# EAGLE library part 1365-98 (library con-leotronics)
DUAL ROW STRAIGHT HEADER 1364 SERIES. 1.27mm x 1.27mm. Without Fixing Post. SMT Source: http://www.leotronics.co.uk/Conexcon/Data%20Sheets/sec.%20A/1364ing.pdf
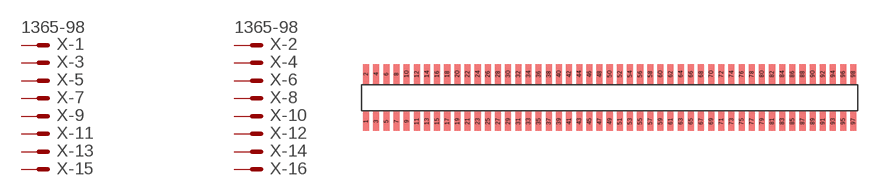
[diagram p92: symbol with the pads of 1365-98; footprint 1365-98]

Designator prefix X; gates -1=MVAL -2=MVAL -3=M -4=M -5=M -6=M -7=M -8=M -9=M -10=M -11=M -12=M -13=M -14=M -15=M -16=M -17=M -18=M -19=M -20=M -21=M -22=M -23=M -24=M -25=M -26=M -27=M -28=M -29=M -30=M -31=M -32=M -33=M -34=M -35=M -36=M -37=M -38=M -39=M -40=M -41=M -42=M -43=M -44=M -45=M -46=M -47=M -48=M -49=M -50=M -51=M -52=M -53=M -54=M -55=M -56=M -57=M -58=M -59=M -60=M -61=M -62=M -63=M -64=M -65=M -66=M -67=M -68=M -69=M -70=M -71=M -72=M -73=M -74=M -75=M -76=M -77=M -78=M -79=M -80=M -81=M -82=M -83=M -84=M -85=M -86=M -87=M -88=M -89=M -90=M -91=M -92=M -93=M -94=M -95=M -96=M -97=M -98=M

## 1365-98 (OC_FARNELL: unknown; OC_NEWARK: unknown)  [1365-98]
1  -1:S  pas
2  -2:S  pas
3  -3:S  pas
4  -4:S  pas
5  -5:S  pas
6  -6:S  pas
7  -7:S  pas
8  -8:S  pas
9  -9:S  pas
10  -10:S  pas
11  -11:S  pas
12  -12:S  pas
13  -13:S  pas
14  -14:S  pas
15  -15:S  pas
16  -16:S  pas
17  -17:S  pas
18  -18:S  pas
19  -19:S  pas
20  -20:S  pas
21  -21:S  pas
22  -22:S  pas
23  -23:S  pas
24  -24:S  pas
25  -25:S  pas
26  -26:S  pas
27  -27:S  pas
28  -28:S  pas
29  -29:S  pas
30  -30:S  pas
31  -31:S  pas
32  -32:S  pas
33  -33:S  pas
34  -34:S  pas
35  -35:S  pas
36  -36:S  pas
37  -37:S  pas
38  -38:S  pas
39  -39:S  pas
40  -40:S  pas
41  -41:S  pas
42  -42:S  pas
43  -43:S  pas
44  -44:S  pas
45  -45:S  pas
46  -46:S  pas
47  -47:S  pas
48  -48:S  pas
49  -49:S  pas
50  -50:S  pas
51  -51:S  pas
52  -52:S  pas
53  -53:S  pas
54  -54:S  pas
55  -55:S  pas
56  -56:S  pas
57  -57:S  pas
58  -58:S  pas
59  -59:S  pas
60  -60:S  pas
61  -61:S  pas
62  -62:S  pas
63  -63:S  pas
64  -64:S  pas
65  -65:S  pas
66  -66:S  pas
67  -67:S  pas
68  -68:S  pas
69  -69:S  pas
70  -70:S  pas
71  -71:S  pas
72  -72:S  pas
73  -73:S  pas
74  -74:S  pas
75  -75:S  pas
76  -76:S  pas
77  -77:S  pas
78  -78:S  pas
79  -79:S  pas
80  -80:S  pas
81  -81:S  pas
82  -82:S  pas
83  -83:S  pas
84  -84:S  pas
85  -85:S  pas
86  -86:S  pas
87  -87:S  pas
88  -88:S  pas
89  -89:S  pas
90  -90:S  pas
91  -91:S  pas
92  -92:S  pas
93  -93:S  pas
94  -94:S  pas
95  -95:S  pas
96  -96:S  pas
97  -97:S  pas
98  -98:S  pas

## Footprint 1365-98 (pad centres in mm)
DUAL ROW STRAIGHT HEADER 1364 SERIES. 1.27mm x 1.27mm. Without Fixing Post. SMT Source: http://www.leotronics.co.uk/Conexcon/Data%20Sheets/sec.%20A/1364ing.pdf
smd 0.76 x 2.4: 1 -30.48,-2.95; 2 -30.48,2.95; 3 -29.21,-2.95; 4 -29.21,2.95; 5 -27.94,-2.95; 6 -27.94,2.95; 7 -26.67,-2.95; 8 -26.67,2.95; 9 -25.4,-2.95; 10 -25.4,2.95; 11 -24.13,-2.95; 12 -24.13,2.95; 13 -22.86,-2.95; 14 -22.86,2.95; 15 -21.59,-2.95; 16 -21.59,2.95; 17 -20.32,-2.95; 18 -20.32,2.95; 19 -19.05,-2.95; 20 -19.05,2.95; 21 -17.78,-2.95; 22 -17.78,2.95; 23 -16.51,-2.95; 24 -16.51,2.95; 25 -15.24,-2.95; 26 -15.24,2.95; 27 -13.97,-2.95; 28 -13.97,2.95; 29 -12.7,-2.95; 30 -12.7,2.95; 31 -11.43,-2.95; 32 -11.43,2.95; 33 -10.16,-2.95; 34 -10.16,2.95; 35 -8.89,-2.95; 36 -8.89,2.95; 37 -7.62,-2.95; 38 -7.62,2.95; 39 -6.35,-2.95; 40 -6.35,2.95; 41 -5.08,-2.95; 42 -5.08,2.95; 43 -3.81,-2.95; 44 -3.81,2.95; 45 -2.54,-2.95; 46 -2.54,2.95; 47 -1.27,-2.95; 48 -1.27,2.95; 49 0,-2.95; 50 0,2.95; 51 1.27,-2.95; 52 1.27,2.95; 53 2.54,-2.95; 54 2.54,2.95; 55 3.81,-2.95; 56 3.81,2.95; 57 5.08,-2.95; 58 5.08,2.95; 59 6.35,-2.95; 60 6.35,2.95; 61 7.62,-2.95; 62 7.62,2.95; 63 8.89,-2.95; 64 8.89,2.95; 65 10.16,-2.95; 66 10.16,2.95; 67 11.43,-2.95; 68 11.43,2.95; 69 12.7,-2.95; 70 12.7,2.95; 71 13.97,-2.95; 72 13.97,2.95; 73 15.24,-2.95; 74 15.24,2.95; 75 16.51,-2.95; 76 16.51,2.95; 77 17.78,-2.95; 78 17.78,2.95; 79 19.05,-2.95; 80 19.05,2.95; 81 20.32,-2.95; 82 20.32,2.95; 83 21.59,-2.95; 84 21.59,2.95; 85 22.86,-2.95; 86 22.86,2.95; 87 24.13,-2.95; 88 24.13,2.95; 89 25.4,-2.95; 90 25.4,2.95; 91 26.67,-2.95; 92 26.67,2.95; 93 27.94,-2.95; 94 27.94,2.95; 95 29.21,-2.95; 96 29.21,2.95; 97 30.48,-2.95; 98 30.48,2.95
